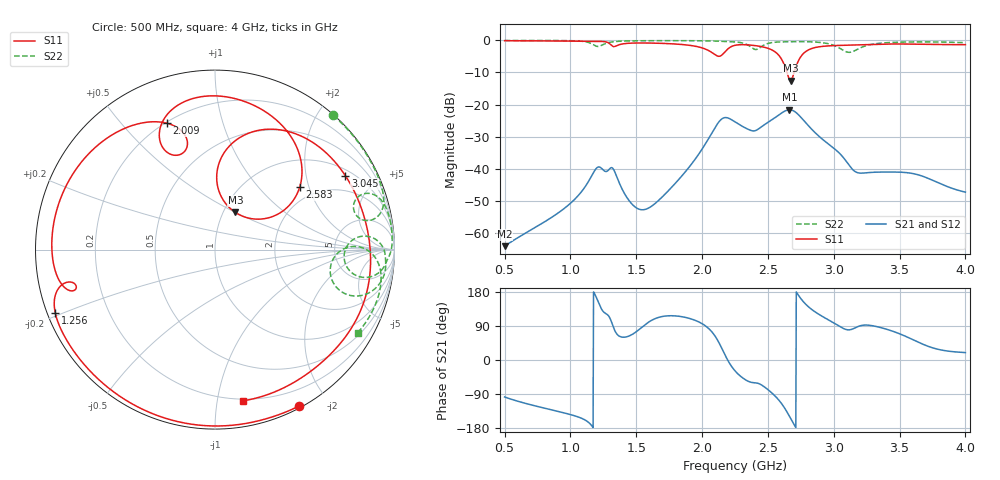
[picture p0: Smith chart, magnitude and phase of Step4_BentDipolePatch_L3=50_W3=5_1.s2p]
! TOUCHSTONE file generated by CST MICROWAVE STUDIO
! Date and time: Tue May 19 14:11:36 2020
! Project name: DualBand_DualMode_Antenna_FD_SteppedDesign.cst
! Parameters = {FPL=20; FPW=20; L=50; ST=10; SW=30; W=52; WF=7; ext=10; gap=1; inset=13}
! Header version: 2015
! Port assignment regex: !\s*Touchstone port\s*([0-9]+)\s*=\s*CST MWS port\s*([0-9]+)\s*\(\"(.*)\"\)(\s*mode\s*([0-9]+))?.*
! Touchstone port assignment:
! Touchstone port 1 = CST MWS port 1 ("")
! Touchstone port 2 = CST MWS port 2 ("")
# GHz S MA R 50
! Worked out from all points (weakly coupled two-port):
!   1006 points, 500 MHz to 4 GHz, reference 50 ohm
!   highest |S21| = -21.64 dB at 2.663 GHz (marker M1); lowest = -64.2 dB at 500 MHz (marker M2)
!   lowest |S11| = -12.5 dB at 2.674 GHz (marker M3), VSWR 1.62, Z = 57 + j25 ohm
!   |S11| at or under -10 dB: 2.644 GHz to 2.699 GHz (54.83 MHz wide, 2.05 % of centre)
!   |S22| runs from -3.7 to 0.0 dB; largest |S21 - S12| = 1.6e-05
!   S11 on the Smith chart (normalised r, x): 500 MHz: 0.02, -1.67; 1.256 GHz: 0.02, -0.19; 2.009 GHz: 0.20, +0.67; 2.583 GHz: 1.64, +1.74; 3.045 GHz: 1.24, +3.38; 4 GHz: 0.19, -1.19
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0.5  0.9886 -61.8  0.0006191 -97.5  0.0006191 -97.5  0.9966 48.6
0.7905  0.9816 -97.6  0.001429 -126.1  0.001428 -126.1  0.9964 28.7
1.0845  0.971 -134.2  0.00439 -153.8  0.004395 -153.8  0.9707 14.8
1.2  0.9679 -149.5  0.01028 162.5  0.01028 162.4  0.8077 14.1
1.256  0.9569 -158.5  0.009266 125.6  0.009262 125.6  0.8772 20.6
1.3225  0.8061 -166.5  0.01008 90.0  0.01008 90.0  0.9501 18.2
1.508  0.9101 177.3  0.002401 76.7  0.002402 76.7  0.9856 11.9
1.669  0.902 156.6  0.003191 112.4  0.003191 112.4  0.9898 8.1
2.0085  0.7541 110.9  0.02147 94.0  0.02147 94.0  0.9847 0.8
2.1415  0.5742 113.6  0.05766 36.7  0.05766 36.7  0.9679 -2.5
2.25  0.8372 102.9  0.05357 -28.5  0.05358 -28.6  0.947 -5.8
2.404  0.8279 73.3  0.03911 -60.2  0.03911 -60.2  0.7215 -3.9
2.5825  0.586 36.4  0.06867 -105.7  0.06867 -105.7  0.9442 -0.6
2.663  0.246 47.5  0.0828 -148.1  0.0828 -148.1  0.9523 -3.5
2.6735  0.2361 61.2  0.08252 -154.8  0.08253 -154.8  0.953 -3.9
2.7295  0.47 87.7  0.07014 172.0  0.07014 172.0  0.9559 -5.7
2.8345  0.7488 63.5  0.04078 132.9  0.04078 132.9  0.9477 -9.8
3.0445  0.8349 29.5  0.01731 88.5  0.01731 88.5  0.7565 -18.6
3.195  0.8522 11.1  0.008546 89.7  0.008546 89.7  0.7525 1.2
3.419  0.8781 -15.3  0.008868 79.3  0.008873 79.2  0.925 -6.4
3.699  0.8647 -47.1  0.007307 38.5  0.007315 38.5  0.9464 -16.5
4  0.8568 -79.4  0.004307 19.6  0.004308 19.6  0.9205 -30.2
